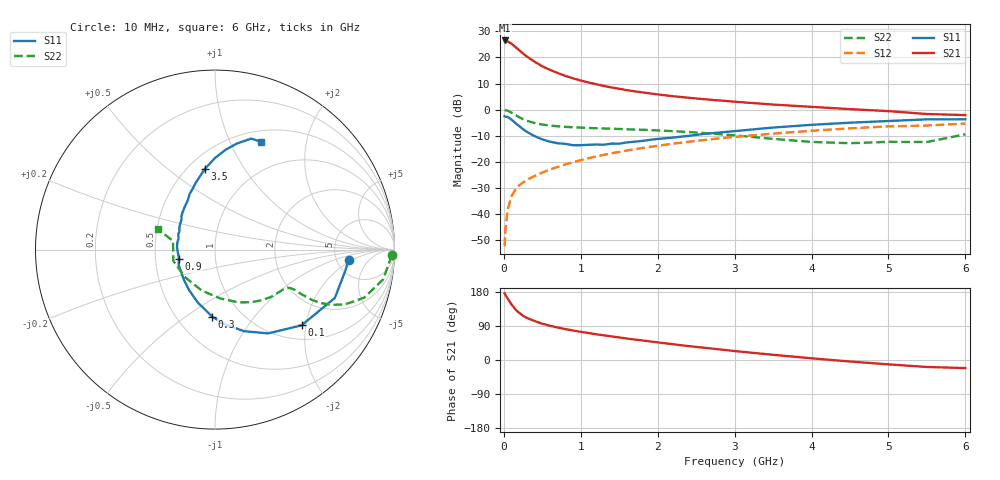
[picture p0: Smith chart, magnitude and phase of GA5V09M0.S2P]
! Infineon Technologies  Discrete & RF Semiconductors
! BF775
! Si NPN RF Bipolar Junction Transistor in SOT23
! VCE = 5 V  IC = 9 mA
! Common Emitter S-Parameters:  May  1996
# GHz  S  MA  R  50
!  f  S11  S21  S12  S22
! GHz  MAG  ANG  MAG  ANG  MAG  ANG  MAG  ANG
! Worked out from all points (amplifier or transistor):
!   36 points, 10 MHz to 6 GHz, reference 50 ohm
!   highest |S21| = 26.5 dB at 10 MHz (marker M1)
!   |S21| within 3 dB of that: start of sweep to 169.8 MHz
!   unconditionally stable (mu >= 1): 633.3 MHz to 3.061 GHz
!   at 250 MHz: K = 0.65, MSG = 24.7 dB, |S12| = -27.9 dB
!   at 1.4 GHz: K = 1.10, MAG = 10.7 dB, |S12| = -16.8 dB
!   at 6 GHz: K = 0.93, MSG = 1.6 dB, |S12| = -5.3 dB
!   S11 on the Smith chart (normalised r, x): 10 MHz: 6.44, -1.66; 100 MHz: 1.32, -1.89; 300 MHz: 0.73, -0.64; 900 MHz: 0.66, -0.07; 3.5 GHz: 0.60, +0.68; 6 GHz: 0.63, +1.31
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0.01  0.7461 -4.4  21.19 176.0  0.0024 87.3  0.9876 -1.9
0.02  0.7364 -8.9  21.08 172.1  0.005 88.2  0.9738 -4.1
0.05  0.7201 -22.0  20.38 161.9  0.012 78.5  0.952 -10.0
0.1  0.6406 -41.2  18.33 146.6  0.0218 71.4  0.8741 -17.8
0.15  0.553 -57.6  15.91 133.5  0.0291 66.2  0.7857 -22.9
0.2  0.4826 -70.4  13.72 124.4  0.0353 63.5  0.7142 -25.5
0.25  0.4199 -82.5  11.89 116.7  0.0401 61.8  0.6557 -26.9
0.3  0.3742 -92.3  10.42 110.9  0.0449 61.8  0.6099 -27.4
0.4  0.3099 -108.0  8.272 102.8  0.0534 62.4  0.552 -27.3
0.5  0.2679 -122.7  6.767 95.7  0.0619 62.7  0.5166 -27.1
0.6  0.2425 -135.2  5.781 90.4  0.071 63.6  0.4937 -26.8
0.7  0.2265 -146.8  5.031 85.7  0.0794 64.4  0.4786 -26.9
0.9  0.2071 -165.4  3.97 77.8  0.0983 64.3  0.4578 -27.8
1.1  0.2113 177.1  3.319 71.2  0.1166 64.2  0.445 -29.7
1.3  0.2119 163.4  2.843 65.1  0.1356 63.2  0.4342 -31.8
1.6  0.2345 147.7  2.356 56.6  0.164 61.3  0.4191 -36.0
2.2  0.2908 125.6  1.804 41.6  0.222 56.4  0.3858 -46.6
2.8  0.3632 109.8  1.498 28.1  0.2804 50.1  0.338 -60.4
3.5  0.4524 97.3  1.249 13.7  0.3461 41.9  0.2743 -83.7
4.5  0.5605 83.8  1.021 -4.0  0.4372 29.1  0.2265 -136.7
5.5  0.6509 71.9  0.822 -18.4  0.4943 14.2  0.2388 168.3
6  0.6525 66.9  0.785 -21.3  0.5417 10.2  0.3355 160.5
